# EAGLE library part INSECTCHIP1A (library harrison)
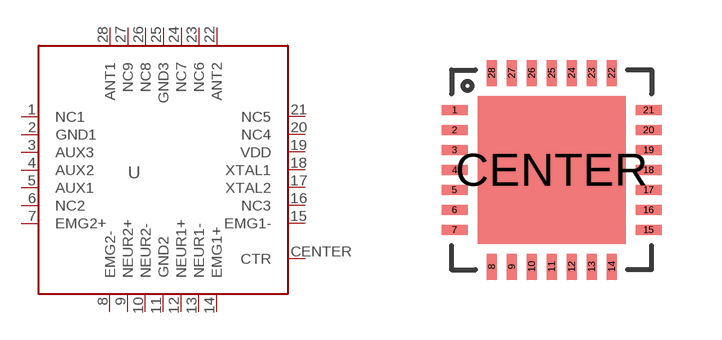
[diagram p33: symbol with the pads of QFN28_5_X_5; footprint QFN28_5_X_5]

Designator prefix U

## INSECTCHIP1A  [QFN28_5_X_5]
1  NC1
2  GND1
3  AUX3
4  AUX2
5  AUX1
6  NC2
7  EMG2+
8  EMG2-
9  NEUR2+
10  NEUR2-
11  GND2
12  NEUR1+
13  NEUR1-
14  EMG1+
15  EMG1-
16  NC3
17  XTAL2
18  XTAL1
19  VDD
20  NC4
21  NC5
22  ANT2
23  NC6
24  NC7
25  GND3
26  NC8
27  NC9
28  ANT1
CENTER  CTR

## Footprint QFN28_5_X_5 (pad centres in mm)
smd 0.65 x 0.25: 1 -2.425,1.5; 2 -2.425,1; 3 -2.425,0.5; 4 -2.425,0; 5 -2.425,-0.5; 6 -2.425,-1; 7 -2.425,-1.5; 15 2.425,-1.5; 16 2.425,-1; 17 2.425,-0.5; 18 2.425,0; 19 2.425,0.5; 20 2.425,1; 21 2.425,1.5
smd 0.25 x 0.65: 8 -1.5,-2.425; 9 -1,-2.425; 10 -0.5,-2.425; 11 0,-2.425; 12 0.5,-2.425; 13 1,-2.425; 14 1.5,-2.425; 22 1.5,2.425; 23 1,2.425; 24 0.5,2.425; 25 0,2.425; 26 -0.5,2.425; 27 -1,2.425; 28 -1.5,2.425
smd 3.7 x 3.7: CENTER 0,0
